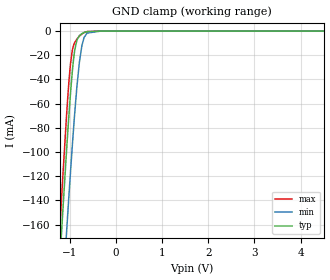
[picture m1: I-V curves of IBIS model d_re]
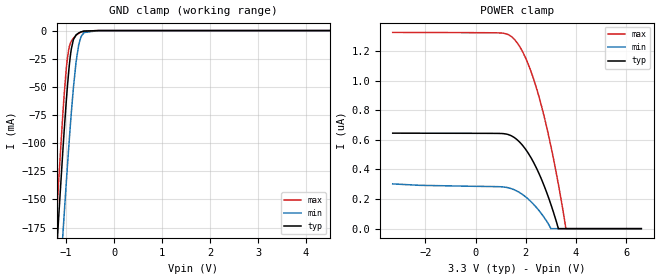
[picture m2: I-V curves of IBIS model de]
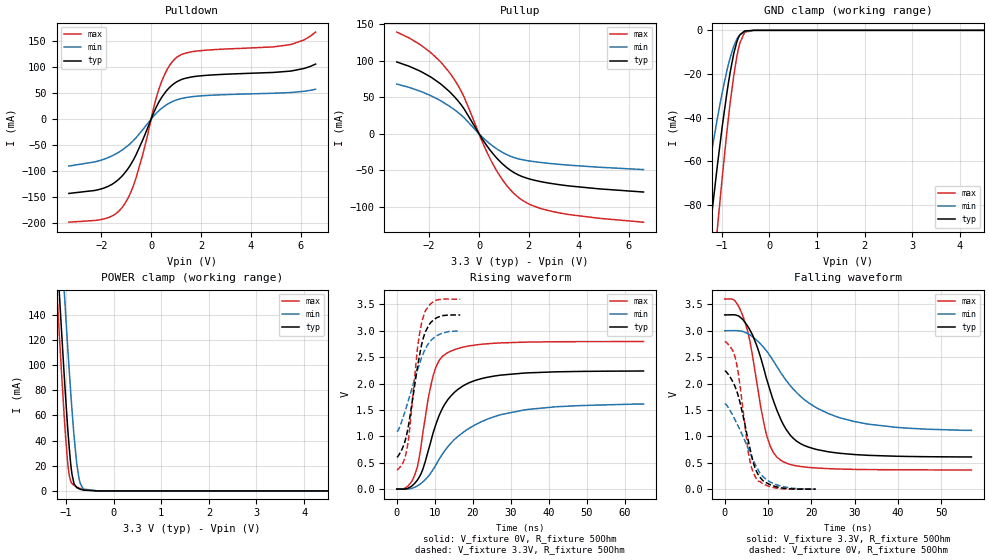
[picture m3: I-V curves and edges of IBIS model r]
|Texas Instruments Incorporated
| SN65HVD7x 3.3-V Supply Full-Duplex RS-485 With IEC ESD Protection
| Marketing part#   Digital Voltage Range   Package-type   #pins
| SN65HVD73DGS   3.0V-3.6V   VSSOP   10
| SN65HVD73DGSR   3.0V-3.6V   VSSOP   10
| SN65HVD73D   3.0V-3.6V   SOIC   14
| SN65HVD73DR   3.0V-3.6V   SOIC   14
[IBIS Ver]   4.1
[File name]   sn65hvd73.ibs
[File Rev]   1.0
[Date]   6/20/2014
[Source]
| Texas Instruments Incorporated.
| Analog-eLab Design Center, HPA
| 12500 TI Blvd
| Dallas, TX -75243
[Notes]   Revision History:
| Rev 1.0: 6/20/2014
| - Initial version of the model
| - Model generated from simulations in TISPICE
| - Model matched to SPICE simulation
| - C_comp although listed in numerical order of value are
|   obtained from varying PVT conditions. For PVT conditions for
|   each specific value refer the buffer description under
|   respective [Model]. IBIS model user is responsible for using
|   appropriate C_comp to simulate for Signal Integrity.
|* EXCEPTION:   *
|* - For model d_re, there is leakage current in the GND   *
|*   clamp I-V Table because of the pullup on pad.   *
|* - For model de, there is leakage current in the POWER   *
|*   clamp I-V Table because of the pulldown on pad.   *
|* - For models a_b_p and a_b_n, there is leakage current in the   *
|*   POWER clamp and GND clamp I-V Table because of the resistor   *
|*   network connected to pad.   *
[Disclaimer]
| This model is designed as an aid for customers of Texas Instruments.
| TI and its licensors and suppliers make no warranties, either expressed
| or implied, with respect to this  model, including the warranties of
| merchantability or fitness for a particular purpose. The model is
| provided solely on an "as is" basis. The entire risk as to its quality
| and performance is with the customer.
[Copyright]
(C) Copyright 2014 Texas Instruments Incorporated.All rights reserved.
|   SN65HVD73DGS
[Component]   SN65HVD73DGS
[Manufacturer]   TI
[Package]   |10 VSSOP  -  DGS package
|   typ   min   max
R_pkg   0.2   0.16   0.24
L_pkg   1.5nH   1.2nH   1.8nH
C_pkg   0.4pF   0.32pF   0.48pF
[Pin]  signal_name   model_name   R_pin   L_pin   C_pin
1   R   r   NA   NA   NA
2   _RE   d_re   NA   NA   NA
3   DE   de   NA   NA   NA
4   D   d_re   NA   NA   NA
5   GND   gnd   NA   NA   NA
6   Y   y_z_p   NA   NA   NA
7   Z   y_z_n   NA   NA   NA
8   B   a_b_n   NA   NA   NA
9   A   a_b_p   NA   NA   NA
10   VCC   power   NA   NA   NA
[Diff_pin]   inv_pin   vdiff   tdelay_typ   tdelay_min   tdelay_max
6   7   NA   0   0   0
9   8   NA   0   0   0
|   SN65HVD73D
[Component]   SN65HVD73D
[Manufacturer]   TI
[Package]   |14 SOIC  -  D package
|   typ   min   max
R_pkg   0.2   0.16   0.24
L_pkg   1.5nH   1.2nH   1.8nH
C_pkg   0.4pF   0.32pF   0.48pF
[Pin]  signal_name   model_name   R_pin   L_pin   C_pin
1   NC   nc   NA   NA   NA
2   R   r   NA   NA   NA
3   _RE   d_re   NA   NA   NA
4   DE   de   NA   NA   NA
5   D   d_re   NA   NA   NA
6   GND   gnd   NA   NA   NA
7   GND   gnd   NA   NA   NA
8   NC   nc   NA   NA   NA
9   Y   y_z_p   NA   NA   NA
10   Z   y_z_n   NA   NA   NA
11   B   a_b_n   NA   NA   NA
12   A   a_b_p   NA   NA   NA
13   VCC   power   NA   NA   NA
14   VCC   power   NA   NA   NA
[Diff_pin]   inv_pin   vdiff   tdelay_typ   tdelay_min   tdelay_max
9   10   NA   0   0   0
12   11   NA   0   0   0
| Models and submodels in the file (7): d_re (Input), de (Input), r (3-state), a_b_p (Input), a_b_n (Input), y_z_p (Output), y_z_n (Output)
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|   d_re Model
[Model]   d_re
Model_type   Input
Vinl = 0.8
Vinh = 2.0
|   typ   min   max
|   (nom PVT)   (fast PVT)   (slow PVT)
C_comp   8.114e-13   7.750e-13   8.695e-13
| Where nom  PVT is Nominal Process, 3.3V, 27C
|   Fast PVT is Strong Process,  3.6V, -40C
|   Slow PVT is Weak Process,   3V, 150C
[Voltage Range]   3.3   3   3.6
|Junction Temperature
[Temperature Range]   27   150   -40
[Power Clamp Reference]   3.3   3   3.6
[GND Clamp Reference]   0   0   0
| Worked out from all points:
|   GND clamp passes 1 mA (typ) near -0.67 V on its own axis
[GND Clamp]
|   Voltage   I(typ)   I(min)   I(max)
-3.3V     -1.706A    -1.709A    -1.74A
-1.33V    -268.5mA   -332.2mA   -244.5mA
-1.176V   -166.3mA   -233.3mA   -138.2mA
-1.064V   -96.82mA   -164.4mA   -67.68mA
-980.1mV  -50.33mA   -115.2mA   -26.33mA
-945.6mV  -34.42mA   -96.08mA   -16.53mA
-891mV    -15.86mA   -67.76mA   -9.449mA
-789mV    -3.689mA   -25.45mA   -4.165mA
-735mV    -2.045mA   -11.84mA   -2.348mA
-686.4mV  -1.144mA   -5.17mA    -1.212mA
-330mV    -1.188uA   -10.17uA   -1.138uA
6.6V      0A         0A         0A
[POWER Clamp]
|   Voltage   I(typ)   I(min)   I(max)
-3.3V     0A         0A         0A
0V        0A         0A         0A
6.6V      0A         0A         0A
|   de Model
[Model]   de
Model_type   Input
Vinl = 0.8
Vinh = 2.0
|   typ   min   max
|   (nom PVT)   (fast PVT)   (slow PVT)
C_comp   8.085e-13   7.723e-13   8.695e-13
| Where nom  PVT is Nominal Process, 3.3V, 27C
|   Fast PVT is Strong Process,  3.6V, -40C
|   Slow PVT is Weak Process,   3V, 150C
[Voltage Range]   3.3   3   3.6
|Junction Temperature
[Temperature Range]   27   150   -40
[Power Clamp Reference]   3.3   3   3.6
[GND Clamp Reference]   0   0   0
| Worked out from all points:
|   GND clamp passes 1 mA (typ) near -0.67 V on its own axis
[GND Clamp]
|   Voltage   I(typ)   I(min)   I(max)
-3.3V     -1.874A    -1.882A    -1.904A
-1.324V   -288.6mA   -359.8mA   -260.8mA
-1.176V   -180.8mA   -255.1mA   -149.1mA
-1.065V   -104.7mA   -179.5mA   -72.15mA
-980.1mV  -53.39mA   -124.8mA   -26.97mA
-945.6mV  -36.1mA    -103.7mA   -16.67mA
-891mV    -16.24mA   -72.63mA   -9.451mA
-792mV    -3.818mA   -27.65mA   -4.283mA
-693mV    -1.245mA   -5.894mA   -1.338mA
-627mV    -485.8uA   -1.777mA   -431.7uA
-330mV    -858.8nA   -10.04uA   -475.9nA
6.6V      0A         0A         0A
[POWER Clamp]
|   Voltage   I(typ)   I(min)   I(max)
-3.3V     644.8nA    302.2nA    1.325uA
933.9mV   643nA      283.5nA    1.322uA
1.412V    628nA      270.8nA    1.299uA
1.729V    588.8nA    246.1nA    1.237uA
1.971V    540.7nA    217.8nA    1.16uA
2.241V    468.8nA    176.7nA    1.045uA
2.507V    379nA      126nA      901.4nA
2.76V     276.3nA    68.43nA    737nA
2.996V    165nA      0A         559.3nA
3.297V    0A         0A         300.1nA
3.598V    0A         0A         0A
6.6V      0A         0A         0A
|   r Model
[Model]   r
Model_type   3-state
Polarity   Non-Inverting
Vmeas = 1.65
Vref = 0
Cref = 2pF
Rref = 70
|   typ   min   max
|   (nom PVT)   (fast PVT)   (slow PVT)
C_comp   2.588e-12   2.046e-12   2.817e-12
| Where nom  PVT is Nominal Process, 3.3V, 27C
|   Fast PVT is Strong Process,  3.6V, -40C
|   Slow PVT is Weak Process,   3V, 150C
[Voltage Range]   3.3   3   3.6
|Junction Temperature
[Temperature Range]   27   150   -40
[Pullup Reference]   3.3   3   3.6
[Pulldown Reference]   0   0   0
[Power Clamp Reference]   3.3   3   3.6
[GND Clamp Reference]   0   0   0
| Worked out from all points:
|   slope of the pulldown table from 0 to 0.495 V, typ, clamps not added: 10.6 ohm
|   slope of the pullup table from 0 to 0.495 V, typ, clamps not added: 20.2 ohm
|   GND clamp passes 1 mA (typ) near -0.56 V on its own axis
|   POWER clamp passes 1 mA (typ) near -0.67 V on its own axis
|   falling waveform, V_fixture 3.3V, R_fixture 50Ohm: 20-80 % time 6.87ns typ, 12.8ns min, 4.29ns max; typ from 3.3 V to 0.61 V
|   rising waveform, V_fixture 0V, R_fixture 50Ohm: 20-80 % time 7.42ns typ, 13.6ns min, 4.14ns max; typ from 0 V to 2.24 V
|   rising waveform, V_fixture 3.3V, R_fixture 50Ohm: 20-80 % time 3.7ns typ, 5.09ns min, 2.84ns max; typ from 0.607 V to 3.3 V
|   falling waveform, V_fixture 0V, R_fixture 50Ohm: 20-80 % time 3.78ns typ, 5.51ns min, 2.72ns max; typ from 2.24 V to 0 V
[Pulldown]
|   Voltage   I(typ)   I(min)   I(max)
-3.3V     -142.9mA   -90.24mA   -198.2mA
-1.752V   -129.9mA   -74.58mA   -190mA
-1.313V   -116.4mA   -64.07mA   -177.8mA
-1.05V    -103.1mA   -55.56mA   -162.3mA
-592.8mV  -67.39mA   -35.2mA    -111.3mA
114mV     13.41mA    6.499mA    24.02mA
346.5mV   35.66mA    17.65mA    62.34mA
663mV     57.01mA    28.87mA    97.12mA
1.042V    72.13mA    37.29mA    119.3mA
1.821V    82.45mA    44.04mA    130.9mA
5.581V    92.36mA    51.13mA    143.3mA
6.6V      105.9mA    57.57mA    167.4mA
[GND Clamp]
|   Voltage   I(typ)   I(min)   I(max)
-3.3V     -803.1mA   -470.3mA   -1.084A
-1.502V   -143.6mA   -96.84mA   -192.8mA
-1.356V   -113mA     -75.22mA   -155.4mA
-1.206V   -82.91mA   -54.43mA   -117.7mA
-1.093V   -61.63mA   -40.07mA   -90.45mA
-895.2mV  -28.72mA   -18.5mA    -46.5mA
-825mV    -19.08mA   -12.43mA   -33.02mA
-751.2mV  -10.69mA   -7.305mA   -20.87mA
-686.4mV  -5.303mA   -4.059mA   -12.14mA
-625.2mV  -2.182mA   -2.075mA   -5.962mA
-520.8mV  -269.2uA   -497.1uA   -854.5uA
6.6V      0A         0A         0A
[Pullup]
|   Voltage   I(typ)   I(min)   I(max)
-3.3V     98.28mA    68.06mA    139.2mA
-2.782V   92.06mA    63.21mA    130.7mA
-1.98V    78.53mA    52.86mA    112.3mA
-1.175V   57.31mA    37.47mA    83.24mA
-603.9mV  34.27mA    22.05mA    50.6mA
161.7mV   -8.749mA   -5.451mA   -13.35mA
656.7mV   -31.16mA   -19.34mA   -47.56mA
1.128V    -46.6mA    -28.71mA   -71.43mA
1.593V    -56.5mA    -34.39mA   -87.39mA
2.185V    -63.25mA   -37.99mA   -98.76mA
3.231V    -69.71mA   -41.87mA   -108.3mA
6.6V      -79.71mA   -48.99mA   -121mA
[POWER Clamp]
|   Voltage   I(typ)   I(min)   I(max)
-3.3V     1.726A     1.762A     1.723A
-1.273V   245.9mA    312.1mA    214.3mA
-1.14V    156.3mA    223.7mA    123.1mA
-1.036V   90.42mA    157.4mA    57.82mA
-953.7mV  44.13mA    107.5mA    18.25mA
-910.8mV  24.82mA    83.2mA     8.67mA
-874.5mV  13.09mA    63.93mA    5.84mA
-777mV    2.686mA    22.24mA    3.242mA
-729mV    1.724mA    10.13mA    2.356mA
-627mV    626uA      1.45mA     889.8uA
-330mV    1.075uA    8.852uA    372.3nA
6.6V      0A         0A         0A
[Ramp]
R_load = 50
|   typ   min   max
dV/dt_r   1.34256/7.38446e-09   0.966209/1.35443e-08  1.67737/4.13854e-09
dV/dt_f   1.61569/6.86378e-09   1.1409/1.30249e-08   1.94163/4.29016e-09
[Falling Waveform]
V_fixture = 3.3V
V_fixture_min = 3V
V_fixture_max = 3.6V
R_fixture = 50Ohm
|   Time   V(typ)   V(min)   V(max)
0s        3.3V       3V         3.6V
2.315ns   3.301V     3.002V     3.573V
4.31ns    3.2V       2.983V     3.255V
5.83ns    3.014V     2.921V     2.797V
9.725ns   2.076V     2.611V     1.009V
11.41ns   1.639V     2.407V     672.8mV
13ns      1.313V     2.2V       546mV
17.65ns   856.3mV    1.748V     428.5mV
26.75ns   678.5mV    1.349V     380.5mV
57ns      610.1mV    1.114V     364.2mV
[Rising Waveform]
V_fixture = 0V
V_fixture_min = 0V
V_fixture_max = 0V
R_fixture = 50Ohm
|   Time   V(typ)   V(min)   V(max)
0s        1.908nV    301.7nV    275.6pV
2.705ns   9.001mV    -576.3uV   43.23mV
4.785ns   113.4mV    36.79mV    278.6mV
6.78ns    359mV      130.5mV    1.022V
9.56ns    1.06V      370.2mV    2.14V
11.31ns   1.42V      582.8mV    2.453V
13.48ns   1.698V     805.8mV    2.588V
18.92ns   2.01V      1.145V     2.711V
27.45ns   2.16V      1.41V      2.77V
64.99ns   2.238V     1.61V      2.796V
[Rising Waveform]
V_fixture = 3.3V
V_fixture_min = 3V
V_fixture_max = 3.6V
R_fixture = 50Ohm
|   Time   V(typ)   V(min)   V(max)
0s        606.8mV    1.095V     363.9mV
1.755ns   820.5mV    1.377V     515.1mV
2.79ns    1.094V     1.618V     806.8mV
3.505ns   1.387V     1.789V     1.211V
5.405ns   2.288V     2.243V     2.64V
6.21ns    2.616V     2.423V     3.027V
7.31ns    2.934V     2.624V     3.337V
8.915ns   3.153V     2.81V      3.509V
10.64ns   3.251V     2.911V     3.585V
16.72ns   3.299V     2.998V     3.6V
[Falling Waveform]
V_fixture = 0V
V_fixture_min = 0V
V_fixture_max = 0V
R_fixture = 50Ohm
|   Time   V(typ)   V(min)   V(max)
0s        2.238V     1.614V     2.796V
1.81ns    2.044V     1.405V     2.632V
2.65ns    1.888V     1.268V     2.412V
3.525ns   1.645V     1.121V     1.973V
5.4ns     933.5mV    776.2mV    722.4mV
6.18ns    646.8mV    624.7mV    416.7mV
7.365ns   334.6mV    418.9mV    188.7mV
8.985ns   151.7mV    226.7mV    94.37mV
11.72ns   50.31mV    90.48mV    23.57mV
21ns      253.8uV    1.73mV     115.9uV
